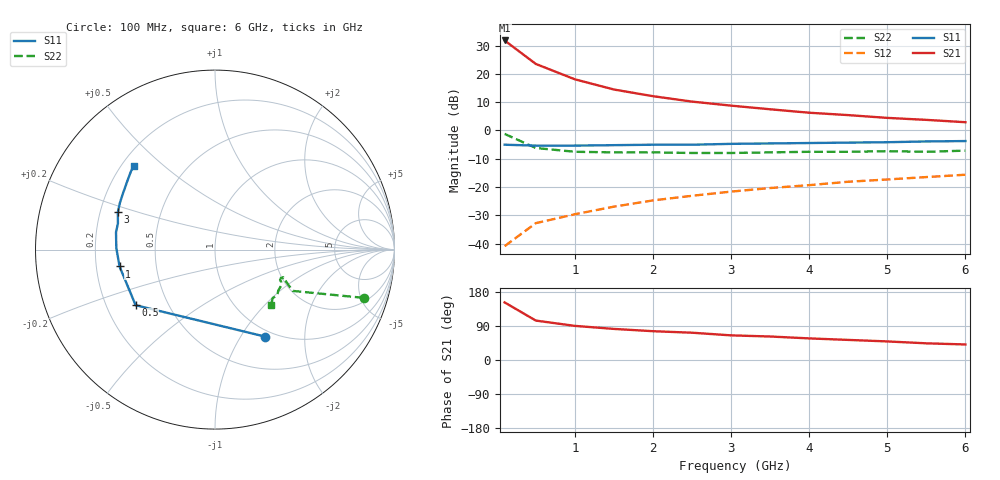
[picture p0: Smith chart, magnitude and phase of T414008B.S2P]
!AT-41400
!S-PARAMETERS at Vce=8V  Ic=25mA.  LAST UPDATED 07-21-92
# ghz s ma r 50
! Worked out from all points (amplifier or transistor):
!   13 points, 100 MHz to 6 GHz, reference 50 ohm
!   highest |S21| = 31.8 dB at 100 MHz (marker M1)
!   |S21| within 3 dB of that: start of sweep to 244.3 MHz
!   unconditionally stable (mu >= 1): 981.5 MHz to 4.49 GHz
!   at 1 GHz: K = 1.01, MAG = 23.2 dB, |S12| = -29.6 dB
!   at 3 GHz: K = 1.11, MAG = 13.2 dB, |S12| = -21.6 dB
!   at 6 GHz: K = 0.89, MSG = 9.3 dB, |S12| = -15.7 dB
!   S11 on the Smith chart (normalised r, x): 100 MHz: 0.91, -1.29; 500 MHz: 0.33, -0.28; 1 GHz: 0.30, -0.08; 3 GHz: 0.27, +0.17; 6 GHz: 0.25, +0.40
0.1  0.56 -60.0  39.07 152.0  0.009 69.0  0.87 -18.0
0.5  0.54 -145.0  15 104.0  0.023 56.0  0.49 -28.0
1  0.54 -170.0  8.03 90.0  0.033 65.0  0.42 -23.0
1.5  0.55 179.0  5.3 82.0  0.045 72.0  0.41 -22.0
2  0.56 170.0  4.04 76.0  0.058 75.0  0.41 -23.0
2.5  0.56 165.0  3.24 72.0  0.07 78.0  0.4 -23.0
3  0.58 159.0  2.75 65.0  0.083 79.0  0.4 -25.0
3.5  0.59 154.0  2.37 62.0  0.096 82.0  0.41 -26.0
4  0.6 149.0  2.06 57.0  0.108 83.0  0.42 -28.0
4.5  0.61 145.0  1.87 53.0  0.124 84.0  0.42 -33.0
5  0.62 142.0  1.67 49.0  0.136 83.0  0.43 -36.0
5.5  0.64 137.0  1.54 44.0  0.15 85.0  0.42 -40.0
6  0.65 134.0  1.4 41.0  0.165 84.0  0.44 -45.0
